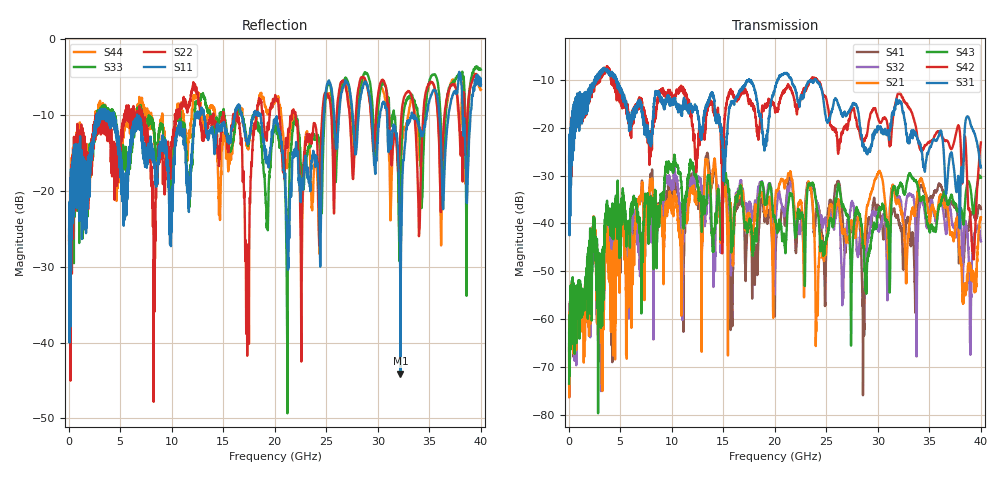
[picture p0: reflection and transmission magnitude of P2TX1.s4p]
!Agilent Technologies,N5245A,MY49151084,A.09.20.08
!Agilent N5245A: A.09.20.08
!Date: Thursday, March 01, 2012 14:00:09
!Correction: S11(Full 4 Port(1,2,3,4))
!S12(Full 4 Port(1,2,3,4))
!S13(Full 4 Port(1,2,3,4))
!S14(Full 4 Port(1,2,3,4))
!S21(Full 4 Port(1,2,3,4))
!S22(Full 4 Port(1,2,3,4))
!S23(Full 4 Port(1,2,3,4))
!S24(Full 4 Port(1,2,3,4))
!S31(Full 4 Port(1,2,3,4))
!S32(Full 4 Port(1,2,3,4))
!S33(Full 4 Port(1,2,3,4))
!S34(Full 4 Port(1,2,3,4))
!S41(Full 4 Port(1,2,3,4))
!S42(Full 4 Port(1,2,3,4))
!S43(Full 4 Port(1,2,3,4))
!S44(Full 4 Port(1,2,3,4))
!S4P File: Measurements: <S11,S12,S13,S14>,
!<S21,S22,S23,S24>,
!<S31,S32,S33,S34>,
!<S41,S42,S43,S44>:
# Hz S  dB  R 50
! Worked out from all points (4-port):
!   3996 points, 50 MHz to 40 GHz, reference 50 ohm
!   strongest paths, dB at 50 MHz, 10.04 GHz, 20.03 GHz, 30.02 GHz, 40 GHz:
!     S31: -27.2, -14.2, -11.5, -20.1, -28.3
!     S42: -26.5, -13.1, -16.6, -17.9, -23.1
!     S43: -73.5, -28.0, -39.3, -38.5, -30.4
!     S21: -66.0, -36.8, -35.7, -29.6, -38.8
!     S32: -62.8, -32.0, -47.1, -41.5, -43.8
!     S41: -65.2, -33.2, -52.9, -36.4, -37.0
!   lowest |S11| = -44.1 dB at 32.2 GHz (marker M1), VSWR 1.01, Z = 49.5 + j0.358 ohm
!   |S11| at or under -10 dB: 6.651 GHz to 12.31 GHz (5.662 GHz wide, 59.7 % of centre); 13.12 GHz to 16.13 GHz (3.005 GHz wide, 20.5 % of centre); 18.62 GHz to 24.77 GHz (6.144 GHz wide, 28.3 % of centre)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
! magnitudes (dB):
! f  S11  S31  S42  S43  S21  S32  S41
! 50 MHz  -25.1  -27.2  -26.5  -73.5  -66.0  -62.8  -65.2
! 9.58 GHz  -17.3  -14.1  -12.7  -28.5  -36.8  -31.1  -34.3
! 17.33 GHz  -13.4  -10.2  -13.2  -41.9  -40.2  -38.6  -41.3
! 28.87 GHz  -5.7  -25.1  -21.9  -52.6  -38.2  -47.4  -44.5
! 32.2 GHz  -44.1  -14.5  -13.0  -31.5  -36.7  -35.0  -40.6
! 39.24 GHz  -7.0  -20.5  -46.2  -37.5  -51.1  -43.8  -37.8
! 40 GHz  -6.1  -28.3  -23.1  -30.4  -38.8  -43.8  -37.0
